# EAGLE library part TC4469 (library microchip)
Logic-Input CMOS Quad Drivers Source: TC 4469-MOSFET-DRIVER.pdf
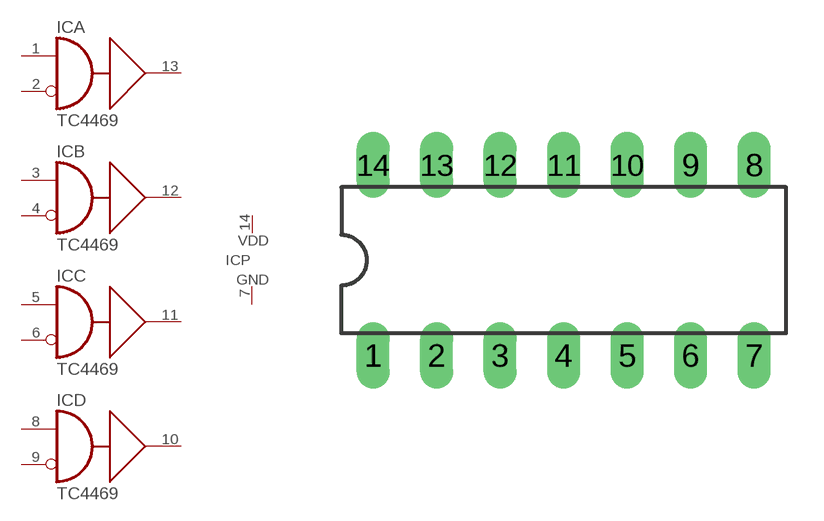
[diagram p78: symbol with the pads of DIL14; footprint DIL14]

Designator prefix IC; gates A=TC4469 B=TC4469 C=TC4469 D=TC4469 P=VDD-GND

## TC4469DP (MF: MICROCHIP; MPN: TC4469CPD; OC_FARNELL: 1439739; OC_NEWARK: 92C6160)  [DIL14]
1  A:A  in
2  A:B  in
3  B:A  in
4  B:B  in
5  C:A  in
6  C:B  in
7  P:GND  pwr
8  D:A  in
9  D:B  in
10  D:Y  out
11  C:Y  out
12  B:Y  out
13  A:Y  out
14  P:VDD  pwr

## TC4469JD (OC_FARNELL: unknown; OC_NEWARK: unknown)  [DIL14]
Pads as for DIL14

## Footprint DIL14 (pad centres in mm)
Dual In Line Package
drill 0.813 long: 1 -7.62,-3.81; 2 -5.08,-3.81; 3 -2.54,-3.81; 4 0,-3.81; 5 2.54,-3.81; 6 5.08,-3.81; 7 7.62,-3.81; 8 7.62,3.81; 9 5.08,3.81; 10 2.54,3.81; 11 0,3.81; 12 -2.54,3.81; 13 -5.08,3.81; 14 -7.62,3.81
